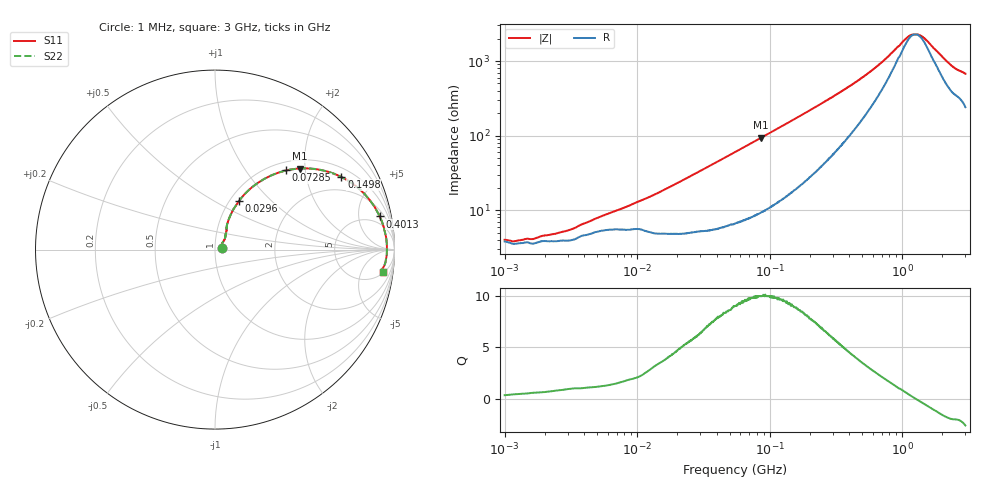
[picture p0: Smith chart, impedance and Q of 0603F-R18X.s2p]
!s-Parameter Generated by FASTRON Sdn. Bhd.
!FASTRON P/N : 0603F-R18X
!Keysight Technologies: E4991B_MY54100416_A.01.15
!Date: Thu Jun 20 13:10:31 2024
!Version  :Rev00  Thu Jun 20 13:10:31 2024
!Data & Calibration Information:
!Freq  S11  S21  S12  S22
!PortZ  Port1:50+j0  Port2:50+j0
!When reading reference impedance value at option line is always used.
! Remarks : This data is being provided solely for informational purposes.
# Hz S dB R 50
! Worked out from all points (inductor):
!   1601 points, 1 MHz to 3 GHz, reference 50 ohm
!   read as one part in series: L = 180 nH near 13.03 MHz
!   highest Q = 10 at 86.36 MHz (marker M1), where L = 172 nH
!   self-resonance near 1.262 GHz
!   S11 on the Smith chart (normalised r, x): 1 MHz: 1.08, +0.03; 29.6 MHz: 1.10, +0.66; 72.85 MHz: 1.16, +1.58; 149.8 MHz: 1.36, +3.22; 401.3 MHz: 3.02, +9.02; 3 GHz: 6, -13
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1000000  -28.30 17.7  -0.32 -0.7  -0.32 -0.7  -28.30 17.7
1179548  -28.70 22.0  -0.30 -0.8  -0.30 -0.8  -28.70 22.0
1649378  -28.10 28.8  -0.30 -1.1  -0.30 -1.1  -28.10 28.8
3037040  -25.80 41.3  -0.34 -2.0  -0.34 -2.0  -25.80 41.3
3804036  -24.20 42.9  -0.39 -2.5  -0.39 -2.5  -24.20 42.9
7898269  -19.90 54.3  -0.50 -5.0  -0.50 -5.0  -19.90 54.3
1.447069e7  -15.80 64.7  -0.52 -8.9  -0.52 -8.9  -15.80 64.7
2.959763e7  -10.40 63.7  -0.84 -17.3  -0.84 -17.3  -10.40 63.7
4.07701e7  -8.11 59.9  -1.19 -23.0  -1.19 -23.0  -8.11 59.9
5.504702e7  -6.14 54.4  -1.75 -29.3  -1.75 -29.3  -6.14 54.4
7.285059e7  -4.54 48.1  -2.53 -36.1  -2.53 -36.1  -4.54 48.1
8.636184e7  -3.71 43.8  -3.15 -40.5  -3.15 -40.5  -3.71 43.8
1.497525e8  -1.81 29.9  -6.00 -53.8  -6.00 -53.8  -1.81 29.9
2.083556e8  -1.17 22.5  -8.27 -60.1  -8.27 -60.1  -1.17 22.5
4.013235e8  -0.57 11.4  -13.80 -66.0  -13.80 -66.0  -0.57 11.4
5.725215e8  -0.45 7.2  -17.60 -64.0  -17.60 -64.0  -0.45 7.2
7.925923e8  -0.39 4.0  -21.80 -55.1  -21.80 -55.1  -0.39 4.0
1.113852e9  -0.37 1.0  -26.90 -22.6  -26.90 -22.6  -0.37 1.0
1.307284e9  -0.37 -0.3  -27.50 6.5  -27.50 6.5  -0.37 -0.3
1.481494e9  -0.37 -1.3  -26.40 28.0  -26.40 28.0  -0.37 -1.3
2.39512e9  -0.49 -5.7  -19.10 57.8  -19.10 57.8  -0.49 -5.7
3e9  -0.52 -7.5  -17.10 61.6  -17.10 61.6  -0.52 -7.5
